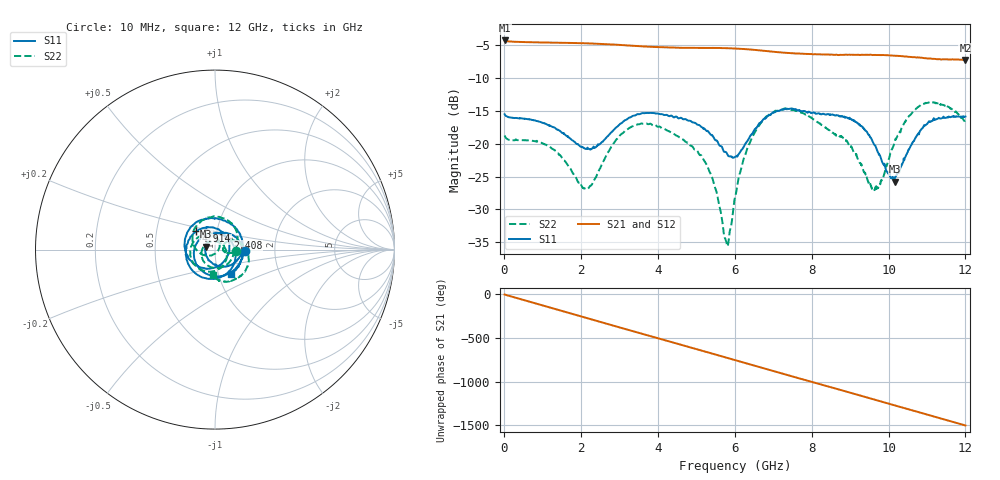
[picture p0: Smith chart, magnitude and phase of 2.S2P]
!Agilent Technologies,E5071C,MY46316741,A.11.02
!Date: Wed Sep 16 11:43:58 2020
!Data & Calibration Information:
!Freq	S11:SOLT2(ON)	S21:SOLT2(ON)	S12:SOLT2(ON)	S22:SOLT2(ON)
!PortZ  Port1:50+j0  Port2:50+j0
!Above PortZ is port z conversion or system Z0 setting when saving the data.
!When reading, reference impedance value at option line is always used.
# Hz S dB R 50
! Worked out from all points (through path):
!   1561 points, 10 MHz to 12 GHz, reference 50 ohm
!   highest |S21| = -4.29 dB at 10 MHz (marker M1); lowest = -7.2 dB at 12 GHz (marker M2)
!   group delay of S21, straight-line fit = 347 ps
!   lowest |S11| = -25.8 dB at 10.16 GHz (marker M3), VSWR 1.11, Z = 45.3 + j1.41 ohm
!   |S11| at or under -10 dB: start of sweep to end of sweep
!   |S22| runs from -35.6 to -13.7 dB; largest |S21 - S12| = 0.0041
!   S11 on the Smith chart (normalised r, x): 10 MHz: 1.40, -0.02; 2.408 GHz: 1.14, +0.15; 4.914 GHz: 0.80, +0.17; 12 GHz: 1.14, -0.32
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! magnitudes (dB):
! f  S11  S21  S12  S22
! 10 MHz  -15.5  -4.3  -4.3  -18.7
! 1.209 GHz  -17.3  -4.6  -4.6  -20.6
! 2.016 GHz  -20.5  -4.7  -4.7  -26.4
! 2.408 GHz  -20.4  -4.8  -4.8  -24.8
! 3.161 GHz  -16.4  -5.0  -5.0  -18.0
! 4.007 GHz  -15.4  -5.3  -5.3  -17.4
! 4.914 GHz  -16.8  -5.4  -5.4  -20.6
! 5.405 GHz  -18.8  -5.4  -5.4  -25.1
! 5.782 GHz  -21.4  -5.5  -5.5  -35.0
! 5.859 GHz  -21.9  -5.5  -5.5  -33.8
! 6.005 GHz  -22.0  -5.5  -5.5  -28.1
! 6.32 GHz  -19.7  -5.6  -5.6  -20.8
! 6.781 GHz  -16.2  -5.9  -5.9  -16.1
! 7.319 GHz  -14.7  -6.2  -6.1  -14.7
! 8.011 GHz  -15.3  -6.4  -6.4  -16.1
! 8.918 GHz  -16.0  -6.5  -6.5  -19.7
! 9.602 GHz  -19.9  -6.5  -6.5  -27.0
! 9.779 GHz  -21.8  -6.5  -6.5  -26.1
! 10 GHz  -24.6  -6.5  -6.6  -22.4
! 10.16 GHz  -25.8  -6.6  -6.6  -19.9
! 10.94 GHz  -17.2  -7.0  -7.0  -13.9
! 12 GHz  -15.9  -7.2  -7.2  -16.9
